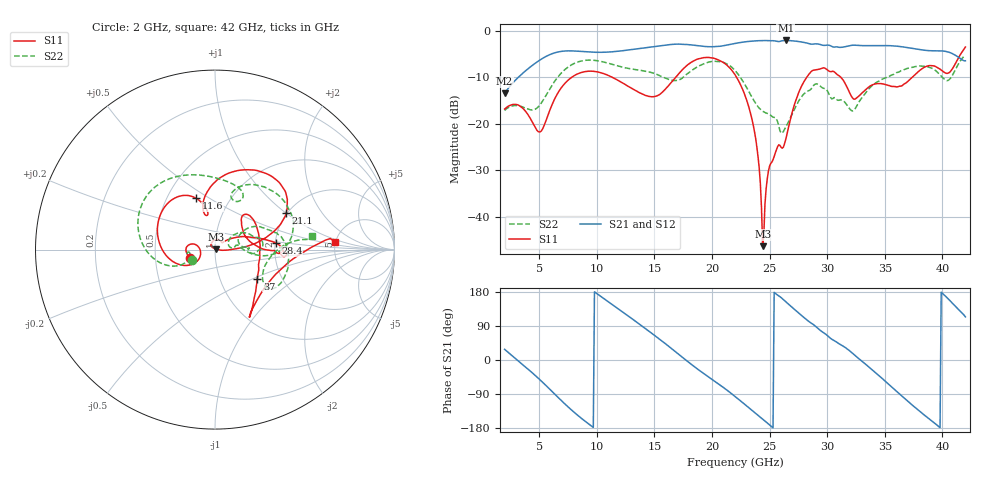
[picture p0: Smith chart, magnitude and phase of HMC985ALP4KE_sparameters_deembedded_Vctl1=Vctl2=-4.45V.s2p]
!s2p File: Measurements: S11, S21, S12, S22
# GHz S dB R 50.0
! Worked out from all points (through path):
!   401 points, 2 GHz to 42 GHz, reference 50 ohm
!   highest |S21| = -2.06 dB at 26.4 GHz (marker M1); lowest = -13.4 dB at 2 GHz (marker M2)
!   lowest |S11| = -46.3 dB at 24.4 GHz (marker M3), VSWR 1.01, Z = 50.4 + j0.222 ohm
!   |S11| at or under -10 dB: start of sweep to 7.821 GHz; 22.14 GHz to 28.22 GHz (6.086 GHz wide, 24.2 % of centre); 31.19 GHz to 37.38 GHz (6.193 GHz wide, 18.1 % of centre)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
!   |S22| runs from -22.0 to -5.2 dB; largest |S21 - S12| = 0.00062
!   S11 on the Smith chart (normalised r, x): 2 GHz: 0.76, -0.07; 11.6 GHz: 0.70, +0.44; 21.1 GHz: 1.97, +1.01; 28.4 GHz: 2.01, +0.17; 37 GHz: 1.51, -0.53; 42 GHz: 4.95, +0.73
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2  -16.83 -161.8  -13.44 28.2  -13.44 28.2  -17.13 -155.6
5  -21.76 -173.3  -6.38 -50.2  -6.39 -50.2  -16.12 -160.2
6.3  -14.88 -150.7  -4.77 -88.4  -4.77 -88.4  -11.01 -161.9
8.7  -8.93 150.1  -4.44 -154.7  -4.45 -154.7  -6.46 151.0
11.6  -10.33 110.2  -4.45 140.8  -4.45 140.8  -7.38 103.2
13.6  -13.16 101.3  -3.85 96.9  -3.85 96.9  -8.43 75.4
15.4  -13.78 106.3  -3.25 56.1  -3.25 56.1  -9.55 61.9
17.9  -7.29 79.9  -2.95 -4.0  -2.95 -4.0  -9.15 72.0
21.1  -7.00 27.3  -3.15 -74.9  -3.15 -74.9  -6.89 15.6
22  -9.42 16.8  -2.71 -96.1  -2.71 -96.1  -8.52 0.2
23.6  -20.48 0.6  -2.18 -135.9  -2.18 -135.8  -14.83 -4.2
24.4  -46.34 27.2  -2.09 -156.0  -2.09 -156.0  -17.30 7.6
25.1  -28.55 124.3  -2.12 -173.8  -2.12 -173.8  -18.16 11.0
26.4  -23.40 41.6  -2.06 153.9  -2.06 154.0  -20.76 33.3
28.4  -9.39 6.4  -2.73 101.9  -2.73 101.9  -12.87 17.8
28.7  -8.58 1.5  -2.87 95.7  -2.87 95.7  -12.18 16.0
30.7  -9.01 -3.4  -3.46 49.9  -3.46 49.9  -14.41 2.0
32.5  -14.55 33.1  -3.10 9.9  -3.10 9.9  -16.46 28.4
35.4  -11.78 18.5  -3.19 -65.6  -3.19 -65.6  -9.76 19.1
37  -10.88 -34.3  -3.60 -108.7  -3.61 -108.7  -8.06 4.5
39.8  -8.24 -56.9  -4.30 -178.6  -4.30 -178.5  -9.44 -35.4
42  -3.48 3.5  -6.43 113.8  -6.44 113.8  -5.23 8.0
